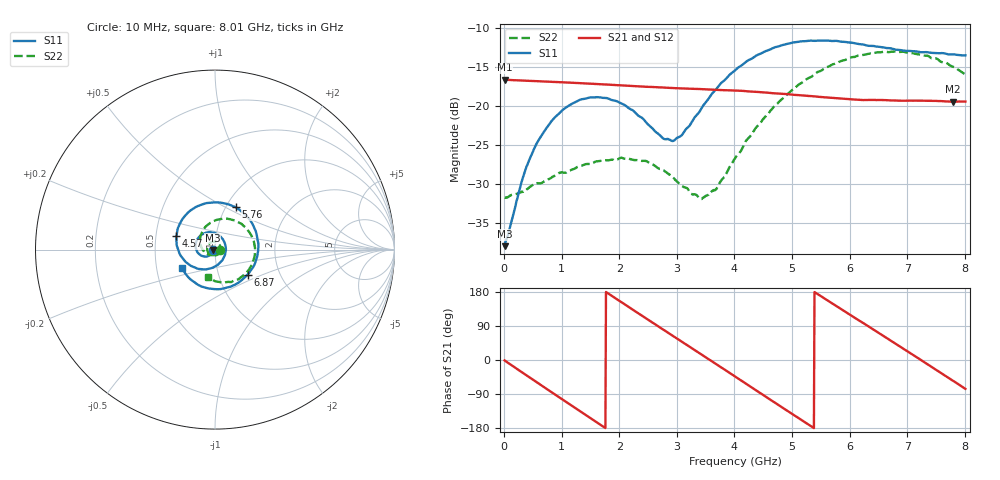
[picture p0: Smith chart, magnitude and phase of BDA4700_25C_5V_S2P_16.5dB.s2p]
!Agilent Technologies,E5071B,MY42404982,A.09.10
!Date: Mon Oct 20 13:34:31 2025
!Data & Calibration Information:
!Freq	S11:SOLT2(ON)	S21:SOLT2(ON)	S12:SOLT2(ON)	S22:SOLT2(ON)
# Hz S RI R 50
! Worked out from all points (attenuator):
!   801 points, 10 MHz to 8.01 GHz, reference 50 ohm
!   highest |S21| = -16.60 dB at 10 MHz (marker M1); lowest = -19.4 dB at 7.79 GHz (marker M2)
!   lowest |S11| = -38.0 dB at 10 MHz (marker M3), VSWR 1.03, Z = 48.8 - j0.158 ohm
!   |S11| at or under -10 dB: start of sweep to end of sweep
!   |S22| runs from -31.9 to -13.0 dB; largest |S21 - S12| = 0.0011
!   S11 on the Smith chart (normalised r, x): 10 MHz: 0.98, -0.00; 4.57 GHz: 0.64, +0.10; 5.76 GHz: 1.11, +0.56; 6.87 GHz: 1.38, -0.40; 8.01 GHz: 0.68, -0.15
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1e7  -0.0125 -0.00162  0.1479 -0.00322  0.1479 -0.00334  0.0258 -0.000871
3.5e8  -0.0245 -0.0276  0.1173 -0.0865  0.1172 -0.0865  0.0221 -0.0178
5.7e8  -0.0432 -0.0384  0.0747 -0.1238  0.0746 -0.1238  0.0141 -0.0287
8.8e8  -0.0777 -0.0332  -0.00125 -0.1429  -0.00125 -0.143  -0.00764 -0.0349
1.35e9  -0.1089 0.0201  -0.1044 -0.0935  -0.1045 -0.0935  -0.0379 -0.0168
1.97e9  -0.0514 0.0938  -0.1275 0.0481  -0.1276 0.0482  -0.033 0.0312
2.45e9  0.0284 0.0747  -0.0486 0.1239  -0.0487 0.1241  0.00155 0.0446
2.68e9  0.0537 0.0387  0.00316 0.132  0.00324 0.132  0.0176 0.0358
2.96e9  0.0577 -0.0176  0.0634 0.1139  0.0635 0.1139  0.0286 0.0185
3.43e9  -0.00567 -0.097  0.1246 0.0317  0.1246 0.0316  0.0176 -0.0181
3.69e9  -0.0686 -0.1097  0.1246 -0.0253  0.1247 -0.0257  -0.00306 -0.0293
4.01e9  -0.1497 -0.0794  0.0915 -0.0865  0.0914 -0.0864  -0.0371 -0.0272
4.57e9  -0.2149 0.074  -0.0201 -0.1204  -0.0199 -0.1204  -0.0815 0.0333
4.92e9  -0.1704 0.1841  -0.0833 -0.0855  -0.0831 -0.0858  -0.0741 0.0935
5.35e9  -0.0373 0.2602  -0.1155 -0.00666  -0.1156 -0.00698  -0.0129 0.155
5.76e9  0.1156 0.2355  -0.0901 0.0673  -0.0901 0.0674  0.0815 0.1699
6.22e9  0.2275 0.1009  -0.0172 0.108  -0.0162 0.1084  0.1831 0.1082
6.68e9  0.223 -0.0762  0.0636 0.0884  0.0638 0.0884  0.2217 -0.0105
6.87e9  0.1822 -0.1391  0.0877 0.0636  0.0879 0.0631  0.2131 -0.0642
7.33e9  0.0268 -0.2205  0.1068 -0.0169  0.1069 -0.0171  0.1347 -0.1626
7.79e9  -0.1361 -0.1663  0.0623 -0.0866  0.0622 -0.0868  0.0122 -0.1788
8.01e9  -0.1846 -0.1036  0.0255 -0.1038  0.0257 -0.1038  -0.0386 -0.154
